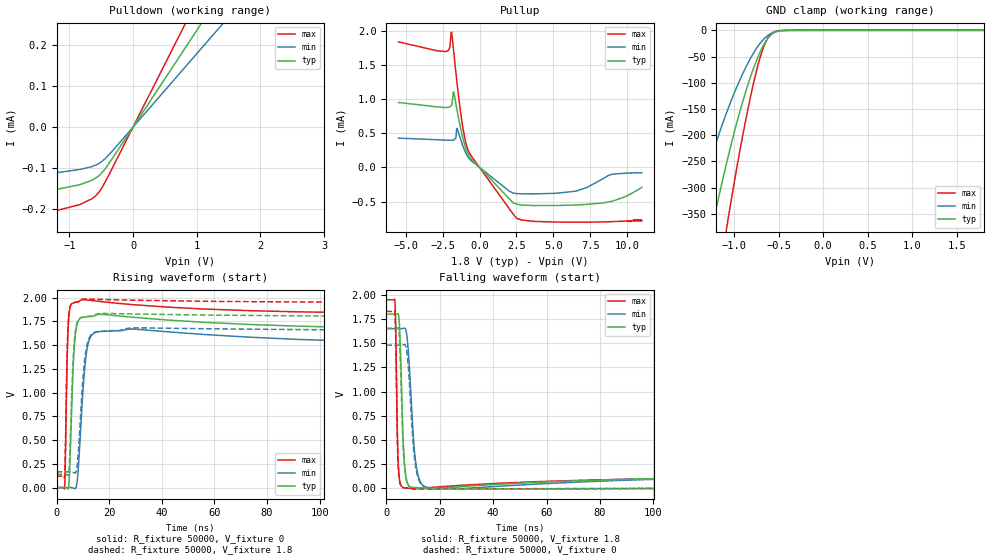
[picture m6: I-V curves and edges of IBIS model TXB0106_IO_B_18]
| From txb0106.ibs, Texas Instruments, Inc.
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[Model]   TXB0106_IO_B_18
Model_type  I/O
Vinl=0.5775
Vinh=1.2675
Enable   Active-High
Vref =   0
Rref =   1e6
Cref =   15p
Vmeas =   0.9
| variable   typ   min   max
C_comp   14.62pF   12.52pF   15.88pF
| C_pullup   14.51pF   12.48pF   15.73pF
| C_pulldown   18.71pF   12.48pF   40.20pF
| C_tri-state   14.62pF   12.52pF   15.88pF
[Temperature Range]   40   100   -40
| Ambient temperature   25   85   -40
[Voltage range]   1.8   1.65   1.95
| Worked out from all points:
|   slope of the pulldown table from 0 to 0.27 V, typ, clamps not added: 4.25 kohm
|   slope of the pullup table from 0 to 0.27 V, typ, clamps not added: 4.38 kohm
|   GND clamp passes 1 mA (typ) near -0.48 V on its own axis
|   rising waveform, R_fixture 50000, V_fixture 0: 20-80 % time 1.24ns typ, 2.01ns min, 728ps max; typ from 0 V to 1.66 V
|   falling waveform, R_fixture 50000, V_fixture 1.8: 20-80 % time 1.12ns typ, 1.95ns min, 645ps max; typ from 1.8 V to 0.134 V
|   rising waveform, R_fixture 50000, V_fixture 1.8: 20-80 % time 1.38ns typ, 2.26ns min, 791ps max; typ from 0.141 V to 1.8 V
|   falling waveform, R_fixture 50000, V_fixture 0: 20-80 % time 1.25ns typ, 2.19ns min, 702ps max; typ from 1.66 V to 0 V
[GND Clamp]
| TXB0104_IO_B_18
|   Voltage   I(typ)   I(min)   I(max)
-5.5V     -5.138A    -3.9A      -6.438A
-1.5V     -595.4mA   -384.3mA   -865.4mA
-1.45V    -550.4mA   -353.7mA   -803.4mA
-1.24V    -372.4mA   -234.8mA   -552.4mA
-1.08V    -251.6mA   -156.2mA   -375.7mA
-1.06V    -237.5mA   -147.2mA   -354.8mA
-920mV    -146.9mA   -89.58mA   -217.5mA
-770mV    -67.75mA   -40.47mA   -93.41mA
-670mV    -28.95mA   -17.51mA   -33.16mA
-575mV    -7.484mA   -5.152mA   -5.709mA
-375mV    -60.21uA   -78.38uA   -9.081uA
1.8V      497pA      3.5nA      55.81pA
[Pulldown]
| TXB0104_IO_B_18
|   Voltage   I(typ)   I(min)   I(max)
-5.5V     -199uA     -145uA     -268uA
-4.31V    -191uA     -139uA     -256uA
-3.315V   -180uA     -132uA     -244uA
-1.73V    -161.7uA   -118.1uA   -218uA
-1.205V   -151.8uA   -111uA     -203.3uA
-830mV    -139.9uA   -103uA     -188.2uA
-645mV    -129.3uA   -95.98uA   -174.4uA
-520mV    -116.2uA   -87.09uA   -155.5uA
-440mV    -102.3uA   -77.27uA   -134.6uA
0V        0A         0A         0A
2.875V    676.5uA    513.7uA    882uA
11V       2.568mA    1.86mA     3.363mA
[Pullup]
| TXB0104_IO_B_18
|   Voltage   I(typ)   I(min)   I(max)
-5.5V     951.6uA    429.1uA    1.839mA
-2.285V   876.8uA    399.9uA    1.698mA
-2.04V    886uA      397.9uA    1.743mA
-1.905V   909.9uA    397.7uA    1.983mA
-1.755V   1.106mA    401.4uA    1.7mA
-1.53V    843.2uA    572.2uA    1.238mA
-1.15V    442.2uA    323.6uA    604.1uA
-815mV    211.4uA    161uA      267.6uA
2.515V    -539.4uA   -382.5uA   -745.1uA
6.52V     -550uA     -348uA     -802uA
8.315V    -521uA     -172uA     -798uA
11V       -292uA     -77uA      -780uA
[Ramp]
| TXB0104_IO_B_18
| variable   typ   min   max
dV/dt_r   1.10/1.48E-09   1.01/2.42E-09   1.20/8.47E-10
dV/dt_f   1.09/1.29E-09   0.99/2.28E-09   1.18/7.25E-10
R_load = 50000
[Rising Waveform]
| TXB0104_IO_B_18
R_fixture =   50000
C_fixture =   0
L_fixture =   0
V_fixture =   0
V_fixture_min = 0
V_fixture_max = 0
|   Time   V(typ)   V(min)   V(max)
0s        90.23nV    1.068uV    24.06nV
3.07ns    140.6uV    -9.532uV   3.9mV
4.06ns    -7.539mV   -89.85uV   1.377V
4.595ns   5.673mV    235.8uV    1.771V
6.83ns    1.513V     -11.29mV   1.948V
7.97ns    1.736V     101.4mV    1.954V
9.405ns   1.789V     726mV      1.977V
11.78ns   1.801V     1.485V     1.976V
16.06ns   1.825V     1.643V     1.962V
220ns     1.66V      1.494V     1.83V
[Falling Waveform]
| TXB0104_IO_B_18
R_fixture =   50000
C_fixture =   0
L_fixture =   0
V_fixture =   1.8
V_fixture_min = 1.65
V_fixture_max = 1.95
|   Time   V(typ)   V(min)   V(max)
0s        1.8V       1.65V      1.95V
3.23ns    1.8V       1.65V      1.936V
3.54ns    1.799V     1.65V      1.638V
4.2ns     1.804V     1.65V      506.7mV
4.67ns    1.781V     1.65V      163.8mV
6.495ns   393.3mV    1.654V     5.994mV
7.99ns    49.35mV    1.503V     1.37mV
11.13ns   6.723mV    245.2mV    -4.217mV
15.08ns   -818.8uV   9.784mV    4.482mV
220ns     134.3mV    148.5mV    117.2mV
[Rising Waveform]
| TXB0104_IO_B_18
R_fixture =   50000
C_fixture =   0
L_fixture =   0
V_fixture =   1.8
V_fixture_min = 1.65
V_fixture_max = 1.95
|   Time   V(typ)   V(min)   V(max)
0s        140.8mV    165.6mV    119.2mV
3.065ns   140.9mV    165.6mV    121.1mV
4.02ns    134.2mV    165.5mV    1.411V
4.58ns    143.3mV    165.8mV    1.793V
6.755ns   1.542V     154.8mV    1.95V
7.935ns   1.747V     258.2mV    1.955V
9.44ns    1.792V     903.6mV    1.982V
11.66ns   1.803V     1.512V     1.986V
15.74ns   1.831V     1.645V     1.983V
220ns     1.801V     1.652V     1.95V
[Falling Waveform]
| TXB0104_IO_B_18
R_fixture =   50000
C_fixture =   0
L_fixture =   0
V_fixture =   0
V_fixture_min = 0
V_fixture_max = 0
|   Time   V(typ)   V(min)   V(max)
0s        1.655V     1.48V      1.828V
3.225ns   1.655V     1.48V      1.817V
3.525ns   1.655V     1.48V      1.543V
4.17ns    1.659V     1.48V      478.2mV
4.66ns    1.639V     1.48V      147.8mV
6.435ns   362.9mV    1.483V     5.171mV
7.915ns   46.31mV    1.357V     614.7uV
10.96ns   3.788mV    224.7mV    -8.88mV
14.84ns   -2.465mV   7.639mV    -8.628mV
220ns     -476uV     -1.107mV   -163.8uV
